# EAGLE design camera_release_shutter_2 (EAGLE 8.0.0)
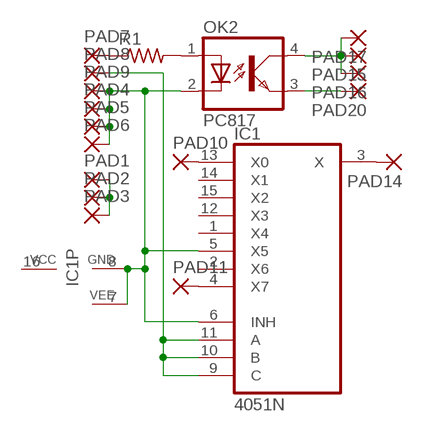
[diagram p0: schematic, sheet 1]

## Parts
IC1  4051N  [DIL16]
OK2  PC817  [DIL04]
PAD1  2,15/1,0  [2,15/1,0]
PAD2  2,15/1,0  [2,15/1,0]
PAD3  2,15/1,0  [2,15/1,0]
PAD4  2,15/1,0  [2,15/1,0]
PAD5  2,15/1,0  [2,15/1,0]
PAD6  2,15/1,0  [2,15/1,0]
PAD7  2,15/1,0  [2,15/1,0]
PAD8  2,15/1,0  [2,15/1,0]
PAD9  2,15/1,0  [2,15/1,0]
PAD10  2,15/1,0  [2,15/1,0]
PAD11  2,15/1,0  [2,15/1,0]
PAD14  2,15/1,0  [2,15/1,0]
PAD15  2,54/1,1  [2,54/1,1]
PAD16  2,54/1,1  [2,54/1,1]
PAD17  2,54/1,1  [2,54/1,1]
PAD20  2,54/1,1  [2,54/1,1]
R1  R-US_0204/7  [0204/7]

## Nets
N$1: OK2.1(A) R1.2
N$2: IC1.9(C) IC1.10(B) IC1.11(A) PAD8.1(P)
N$3: OK2.4(COL) PAD15.1(P) PAD16.1(P) PAD17.1(P)
N$5: IC1.13(X0) PAD10.1(P)
N$6: IC1.4(X7) PAD11.1(P)
N$7: PAD1.1(P) PAD2.1(P) PAD3.1(P)
N$8: OK2.3(EMIT) PAD20.1(P)
N$10: IC1.5(X5) IC1.6(INH) IC1.7(VEE) IC1.8(GND) OK2.2(C) PAD4.1(P) PAD5.1(P) PAD6.1(P) PAD9.1(P)
N$11: IC1.3(X) PAD14.1(P)
N$20: PAD7.1(P) R1.1
Unconnected: IC1.1(X4) IC1.2(X6) IC1.12(X3) IC1.14(X1) IC1.15(X2)

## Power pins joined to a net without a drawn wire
VCC: IC1.16(VCC)

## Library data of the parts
IC1 = 40xx:4051: 8-channel ANALOG MULTIPLEXER
OK2 = optocoupler:PC817: SHARP OPTO COUPLER; MPN: PC817X4J000F; OC_FARNELL: 9707727; OC_NEWARK: 97K7059
PAD1-PAD11 PAD14 = wirepad:2,15/1,0: THROUGH-HOLE PAD
PAD15-PAD17 PAD20 = wirepad:2,54/1,1: THROUGH-HOLE PAD
R1 = resistor:R-US_: RESISTOR, American symbol

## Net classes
0 default: width 0.381 mm, drill 0.406 mm, clearance 0.254 mm

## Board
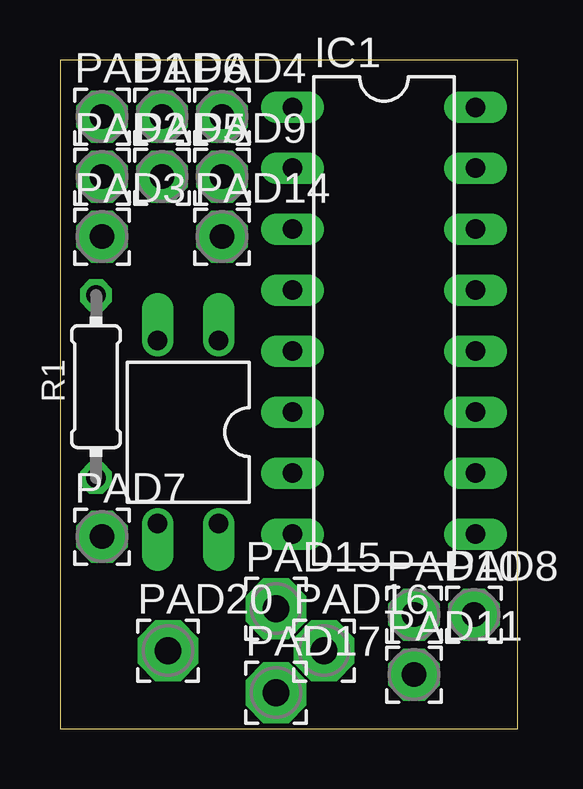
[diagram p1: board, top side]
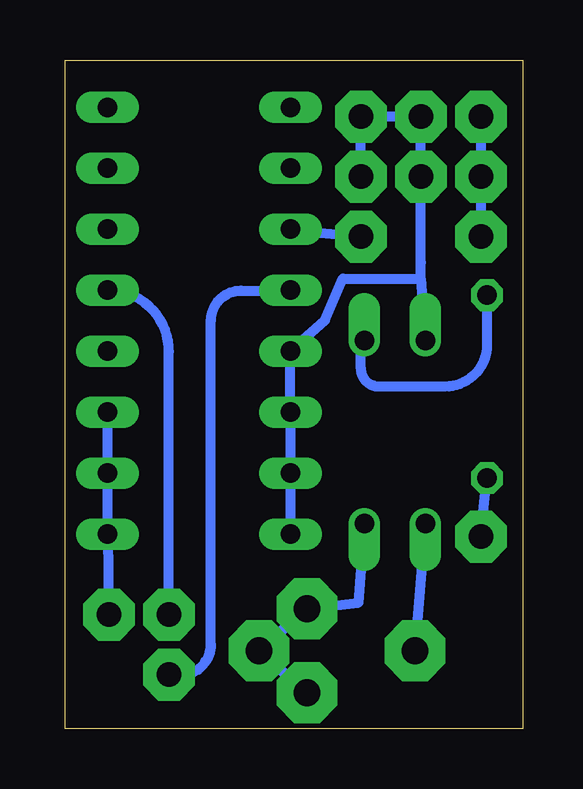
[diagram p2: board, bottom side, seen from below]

Size 19.07 x 27.86 mm. Coordinates in mm from the lower left corner, seen from the top.
Outline: 0,0 19.07,0 19.07,27.86 0,27.86 0,0
Copper layers (1*16): Top 0.035mm / dielectric 1.5mm / Bottom 0.035mm
Design rules "default": minimum track width 10mil, minimum drill 24mil, track to track 8mil, track to pad 8mil, pad to pad 8mil, via to via 8mil, smd to smd 8mil, copper to edge 40mil, drill to drill 8mil, minimum pad ring 10mil, minimum via ring 8mil, stop-mask expansion 4mil, vias tented up to drill 0mil, thermal gap 10mil

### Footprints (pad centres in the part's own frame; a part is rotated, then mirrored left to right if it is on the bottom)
DIL16 = drill 0.813 long: 1 -8.89,-3.81; 2 -6.35,-3.81; 3 -3.81,-3.81; 4 -1.27,-3.81; 5 1.27,-3.81; 6 3.81,-3.81; 7 6.35,-3.81; 8 8.89,-3.81; 9 8.89,3.81; 10 6.35,3.81; 11 3.81,3.81; 12 1.27,3.81; 13 -1.27,3.81; 14 -3.81,3.81; 15 -6.35,3.81; 16 -8.89,3.81
DIL04 = drill 0.813 offset: 1 -1.27,-3.81; 2 1.27,-3.81; 3 1.27,3.81; 4 -1.27,3.81
2,15/1,0 = drill 1.016 pad 2.159 octagon: 1 0,0
2,54/1,1 = drill 1.118 pad 2.54 octagon: 1 0,0
0204/7 = drill 0.813 octagon: 1 -3.81,0; 2 3.81,0

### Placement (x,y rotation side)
IC1  13.5,17 270 top
OK2  5.34,12.36 180 top
PAD1  1.75,25.5 0 top
PAD2  1.75,23 0 top
PAD3  1.75,20.5 0 top
PAD4  6.75,25.5 0 top
PAD5  4.25,23 0 top
PAD6  4.25,25.5 0 top
PAD7  1.75,8 0 top
PAD8  17.25,4.75 0 top
PAD9  6.75,23 0 top
PAD10  14.75,4.75 0 top
PAD11  14.75,2.25 0 top
PAD14  6.75,20.5 0 top
PAD15  9,5 0 top
PAD16  11,3.25 0 top
PAD17  9,1.5 0 top
PAD20  4.5,3.25 0 top
R1  1.5,14.25 90 top

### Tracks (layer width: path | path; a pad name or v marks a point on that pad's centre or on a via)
N$1
  Bottom 0.406: R1.2 1.5,16 arc90 3.25,14.25 6,14.25 arc90 6.75,15 6.75,16.05 arc-90 OK2.1
N$2
  Bottom 0.406: PAD8.1 IC1.9 IC1.10 IC1.11
N$3
  Bottom 0.406: OK2.4 6.86,5.25 PAD15.1 PAD16.1 PAD17.1
N$5
  Bottom 0.406: IC1.13 arc90 14.75,15.71 PAD10.1
N$6
  Bottom 0.406: PAD11.1 14.25,2.25 arc-90 13,3.5 13,17 arc90 11.75,18.25 9.71,18.25 arc-90 IC1.4
N$7
  Bottom 0.406: PAD1.1 PAD2.1 PAD3.1
N$8
  Bottom 0.406: OK2.3 PAD20.1
N$10
  Bottom 0.406: PAD9.1 PAD4.1 PAD6.1 PAD5.1 4.25,19.41 4.26,18.75 | 4.26,18.75 OK2.2 | IC1.8 IC1.7 IC1.6 IC1.5 8.25,17 7.5,18.75 4.26,18.75
N$11
  Bottom 0.406: PAD14.1 9.69,20.75 IC1.3
N$20
  Bottom 0.406: PAD7.1 R1.1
